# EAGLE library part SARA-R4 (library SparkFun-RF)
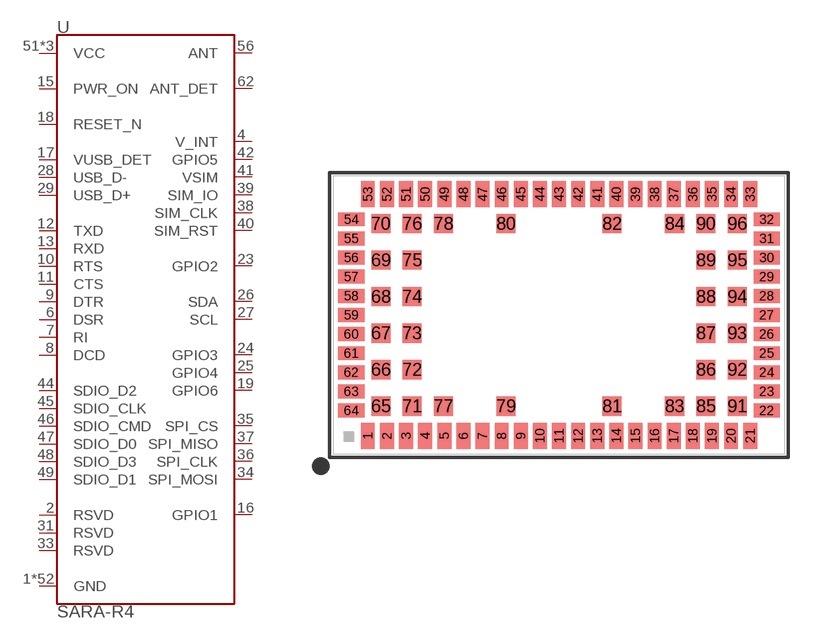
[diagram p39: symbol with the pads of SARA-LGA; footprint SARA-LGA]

Designator prefix U

## SARA-R4 (PROD_ID: IC-14085)  [SARA-LGA]
1  GND
2  RSVD
3  GND
4  V_INT
5  GND
6  DSR
7  RI
8  DCD
9  DTR
10  RTS
11  CTS
12  TXD
13  RXD
14  GND
15  PWR_ON
16  GPIO1
17  VUSB_DET
18  RESET_N
19  GPIO6
20  GND
21  GND
22  GND
23  GPIO2
24  GPIO3
25  GPIO4
26  SDA
27  SCL
28  USB_D-
29  USB_D+
30  GND
31  RSVD
32  GND
33  RSVD
34  SPI_MOSI
35  SPI_CS
36  SPI_CLK
37  SPI_MISO
38  SIM_CLK
39  SIM_IO
40  SIM_RST
41  VSIM
42  GPIO5
43  GND
44  SDIO_D2
45  SDIO_CLK
46  SDIO_CMD
47  SDIO_D0
48  SDIO_D3
49  SDIO_D1
50  GND
51  VCC
52  VCC
53  VCC
54  GND
55  GND
56  ANT
57  GND
58  GND
59  GND
60  GND
61  GND
62  ANT_DET
63  GND
64  GND
65  GND
66  GND
67  GND
68  GND
69  GND
70  GND
71  GND
72  GND
73  GND
74  GND
75  GND
76  GND
77  GND
78  GND
79  GND
80  GND
81  GND
82  GND
83  GND
84  GND
85  GND
86  GND
87  GND
88  GND
89  GND
90  GND
91  GND
92  GND
93  GND
94  GND
95  GND
96  GND

## Footprint SARA-LGA (pad centres in mm)
ublox SARA LGA form factor Miniature cellular modem package. Common form factor for many ublox cellular modules, including SARA-R4 and SARA-U2 series. Dimensions: 26.0 x 16.0 mm Pins: 96 Pitch: 1.1mm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
smd 0.8 x 1.5: 1 -11,-6.95; 2 -9.9,-6.95; 3 -8.8,-6.95; 4 -7.7,-6.95; 5 -6.6,-6.95; 6 -5.5,-6.95; 7 -4.4,-6.95; 8 -3.3,-6.95; 9 -2.2,-6.95; 10 -1.1,-6.95; 11 0,-6.95; 12 1.1,-6.95; 13 2.2,-6.95; 14 3.3,-6.95; 15 4.4,-6.95; 16 5.5,-6.95; 17 6.6,-6.95; 18 7.7,-6.95; 19 8.8,-6.95; 20 9.9,-6.95; 21 11,-6.95; 33 11,6.95; 34 9.9,6.95; 35 8.8,6.95; 36 7.7,6.95; 37 6.6,6.95; 38 5.5,6.95; 39 4.4,6.95; 40 3.3,6.95; 41 2.2,6.95; 42 1.1,6.95; 43 0,6.95; 44 -1.1,6.95; 45 -2.2,6.95; 46 -3.3,6.95; 47 -4.4,6.95; 48 -5.5,6.95; 49 -6.6,6.95; 50 -7.7,6.95; 51 -8.8,6.95; 52 -9.9,6.95; 53 -11,6.95
smd 1.5 x 0.8: 22 11.95,-5.5; 23 11.95,-4.4; 24 11.95,-3.3; 25 11.95,-2.2; 26 11.95,-1.1; 27 11.95,0; 28 11.95,1.1; 29 11.95,2.2; 30 11.95,3.3; 31 11.95,4.4; 32 11.95,5.5; 54 -11.95,5.5; 55 -11.95,4.4; 56 -11.95,3.3; 57 -11.95,2.2; 58 -11.95,1.1; 59 -11.95,0; 60 -11.95,-1.1; 61 -11.95,-2.2; 62 -11.95,-3.3; 63 -11.95,-4.4; 64 -11.95,-5.5
smd 1.1 x 1.1: 65 -10.25,-5.25; 66 -10.25,-3.15; 67 -10.25,-1.05; 68 -10.25,1.05; 69 -10.25,3.15; 70 -10.25,5.25; 71 -8.45,-5.25; 72 -8.45,-3.15; 73 -8.45,-1.05; 74 -8.45,1.05; 75 -8.45,3.15; 76 -8.45,5.25; 77 -6.65,-5.25; 78 -6.65,5.25; 79 -3.05,-5.25; 80 -3.05,5.25; 81 3.05,-5.25; 82 3.05,5.25; 83 6.65,-5.25; 84 6.65,5.25; 85 8.45,-5.25; 86 8.45,-3.15; 87 8.45,-1.05; 88 8.45,1.05; 89 8.45,3.15; 90 8.45,5.25; 91 10.25,-5.25; 92 10.25,-3.15; 93 10.25,-1.05; 94 10.25,1.05; 95 10.25,3.15; 96 10.25,5.25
